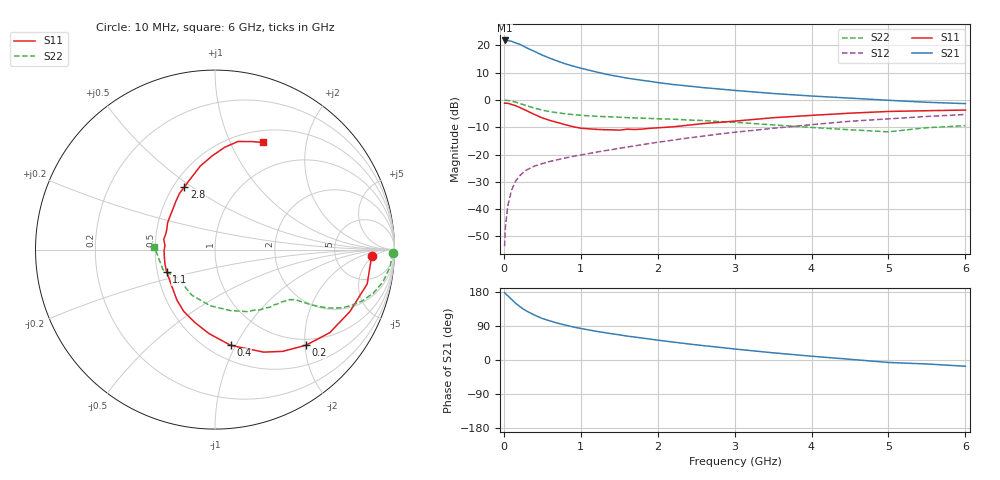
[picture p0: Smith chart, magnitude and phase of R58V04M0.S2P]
! SIEMENS Small Signal Semiconductors
! BFR183
! Si NPN RF Bipolar Junction Transistor in SOT23
! VCE = 8 V  IC = 4 mA
! Common Emitter S-Parameters:  May  1996
# GHz  S  MA  R  50
!  f  S11  S21  S12  S22
! GHz  MAG  ANG  MAG  ANG  MAG  ANG  MAG  ANG
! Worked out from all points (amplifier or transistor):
!   36 points, 10 MHz to 6 GHz, reference 50 ohm
!   highest |S21| = 21.8 dB at 10 MHz (marker M1)
!   |S21| within 3 dB of that: start of sweep to 319.1 MHz
!   unconditionally stable (mu >= 1): 1.179 GHz to 2.728 GHz
!   at 250 MHz: K = 0.36, MSG = 23.2 dB, |S12| = -26.6 dB
!   at 1.4 GHz: K = 1.05, MAG = 12.2 dB, |S12| = -18.2 dB
!   at 6 GHz: K = 0.87, MSG = 2.0 dB, |S12| = -5.3 dB
!   S11 on the Smith chart (normalised r, x): 10 MHz: 13, -4; 200 MHz: 0.87, -2.02; 400 MHz: 0.63, -0.95; 1.1 GHz: 0.56, -0.15; 2.8 GHz: 0.57, +0.47; 6 GHz: 0.64, +1.33
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0.01  0.8728 -2.4  12.29 177.9  0.0021 81.3  0.9905 -1.1
0.02  0.8695 -5.3  12.06 175.6  0.0046 83.7  0.9865 -2.2
0.05  0.8693 -12.7  12.2 169.7  0.0113 83.1  0.9807 -5.6
0.1  0.8274 -24.6  11.88 160.1  0.0222 77.4  0.953 -10.9
0.15  0.7893 -35.9  11.12 150.3  0.0321 70.7  0.9148 -15.4
0.2  0.7351 -46.5  10.57 142.2  0.0401 66.8  0.869 -19.2
0.25  0.6807 -56.4  9.764 134.7  0.0467 62.6  0.8217 -22.2
0.3  0.6324 -64.6  8.952 128.7  0.0527 60.2  0.7822 -24.5
0.4  0.5404 -80.7  7.723 118.5  0.0616 56.5  0.7094 -27.3
0.5  0.4696 -94.0  6.627 109.6  0.0684 54.5  0.65 -29.0
0.6  0.4212 -105.5  5.795 103.1  0.0748 53.6  0.6097 -30.0
0.7  0.3854 -117.0  5.143 97.2  0.0805 53.3  0.5824 -30.6
0.9  0.3237 -136.1  4.169 87.3  0.0928 53.7  0.5391 -31.6
1.1  0.2965 -155.4  3.529 79.5  0.1041 55.1  0.5122 -33.0
1.3  0.2854 -171.0  3.024 72.6  0.1171 55.9  0.4947 -34.5
1.6  0.2913 168.7  2.513 63.2  0.1369 56.5  0.4757 -37.6
2.2  0.3223 137.5  1.92 47.3  0.1837 56.2  0.4449 -46.0
2.8  0.3884 116.0  1.588 33.5  0.2378 53.1  0.4011 -57.3
3.5  0.4725 100.0  1.314 19.0  0.3023 46.8  0.349 -76.3
4.5  0.5726 84.6  1.081 1.9  0.4073 35.6  0.2846 -117.2
5.5  0.6357 71.2  0.907 -10.5  0.4991 23.2  0.3106 -158.8
6  0.6533 66.1  0.857 -16.5  0.5411 15.0  0.3378 177.5
